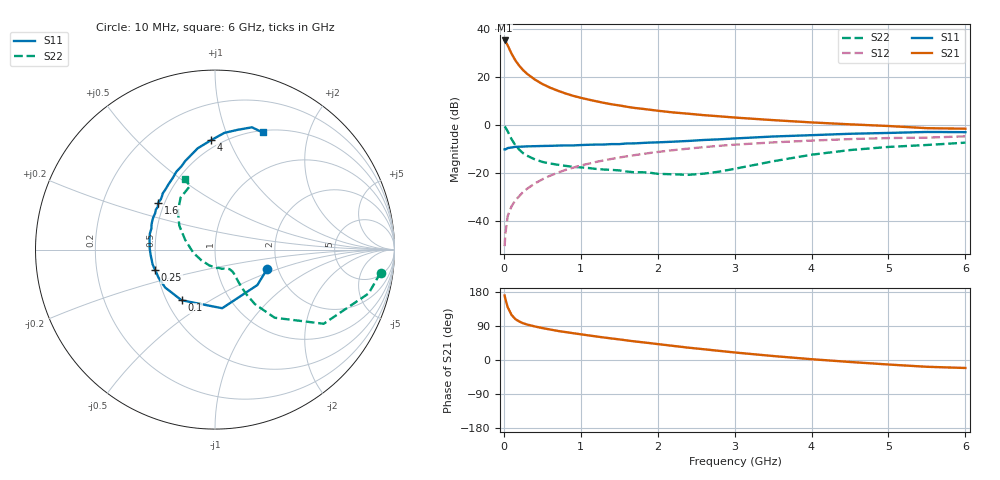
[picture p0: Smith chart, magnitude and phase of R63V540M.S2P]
! SIEMENS Small Signal Semiconductors
! BFR193
! Si NPN RF Bipolar Junction Transistor in SOT23
! VCE = 3.5 V  IC = 40 mA
! Common Emitter S-Parameters:  May  1996
# GHz  S  MA  R  50
!  f  S11  S21  S12  S22
! GHz  MAG  ANG  MAG  ANG  MAG  ANG  MAG  ANG
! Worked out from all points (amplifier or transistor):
!   36 points, 10 MHz to 6 GHz, reference 50 ohm
!   highest |S21| = 35.1 dB at 10 MHz (marker M1)
!   |S21| within 3 dB of that: start of sweep to 63.88 MHz
!   unconditionally stable (mu >= 1): 417.6 MHz to 1.891 GHz
!   at 250 MHz: K = 0.93, MSG = 25.3 dB, |S12| = -27.9 dB
!   at 1.4 GHz: K = 1.02, MAG = 10.5 dB, |S12| = -14.2 dB
!   at 6 GHz: K = 0.95, MSG = 1.6 dB, |S12| = -4.8 dB
!   S11 on the Smith chart (normalised r, x): 10 MHz: 1.75, -0.42; 100 MHz: 0.60, -0.38; 250 MHz: 0.49, -0.13; 1.6 GHz: 0.46, +0.29; 4 GHz: 0.44, +0.86; 6 GHz: 0.52, +1.35
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0.01  0.31 -20.5  56.9 170.2  0.003 82.1  0.9311 -7.9
0.02  0.3077 -39.9  54.82 161.0  0.0054 78.1  0.8905 -15.9
0.05  0.3291 -83.0  44.95 139.3  0.0127 71.3  0.7333 -34.3
0.1  0.3381 -123.4  30.3 119.0  0.0203 67.9  0.5045 -48.8
0.15  0.349 -142.7  21.87 107.9  0.0269 68.9  0.3764 -53.8
0.2  0.3513 -153.3  17 101.6  0.0329 70.5  0.3054 -54.9
0.25  0.3529 -161.2  13.76 97.0  0.0402 71.7  0.2577 -54.8
0.3  0.3572 -166.6  11.6 93.7  0.0466 72.8  0.2292 -54.2
0.4  0.3599 -175.3  8.827 88.7  0.06 73.6  0.1924 -52.9
0.5  0.3636 179.3  7.089 84.3  0.0735 73.5  0.1699 -51.6
0.6  0.3661 174.5  5.95 80.5  0.0875 72.9  0.1573 -51.5
0.8  0.3737 166.4  4.508 73.8  0.1152 70.9  0.1404 -52.9
0.9  0.3733 161.8  4.023 70.7  0.1286 69.9  0.134 -53.8
1.1  0.3855 154.8  3.356 64.9  0.1555 67.8  0.1266 -58.5
1.3  0.3898 148.9  2.867 59.4  0.1827 65.0  0.1178 -63.7
1.6  0.4109 140.4  2.377 51.6  0.2219 60.7  0.1069 -75.6
2.2  0.4465 125.5  1.813 37.3  0.2974 51.9  0.0937 -109.7
3.5  0.5726 99.7  1.254 10.5  0.4317 31.4  0.1748 161.9
4  0.6103 92.0  1.124 2.1  0.4707 24.4  0.2393 146.2
4.5  0.6525 85.4  1.025 -5.2  0.5056 17.3  0.2991 133.7
5.5  0.7117 73.2  0.853 -17.9  0.542 3.5  0.3813 111.3
6  0.7048 67.9  0.832 -21.1  0.577 -0.6  0.4264 113.4
